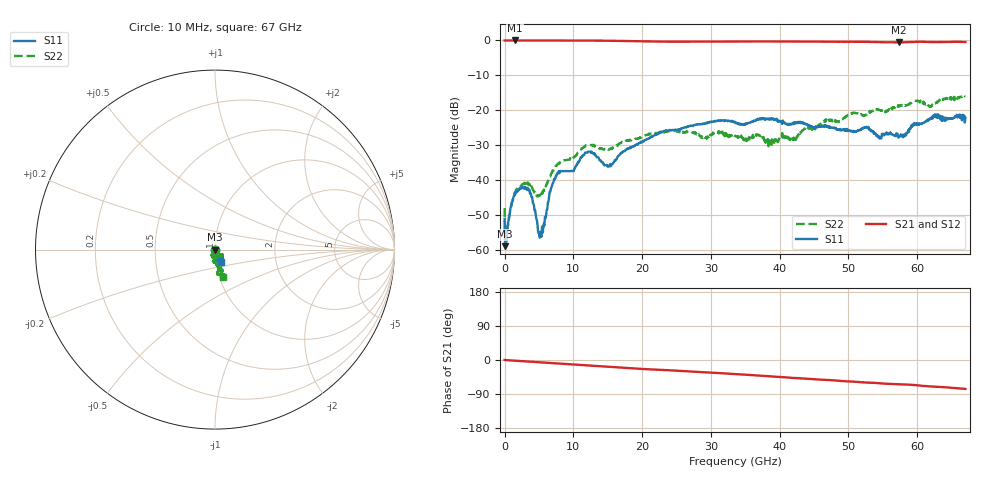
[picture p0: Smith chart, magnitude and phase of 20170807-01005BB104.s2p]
# MHz S RI R 50
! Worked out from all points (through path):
!   801 points, 10 MHz to 67 GHz, reference 50 ohm
!   highest |S21| = 0.00 dB at 1.517 GHz (marker M1); lowest = -0.6 dB at 57.37 GHz (marker M2)
!   group delay of S21, straight-line fit = 3.09 ps
!   lowest |S11| = -59.0 dB at 93.74 MHz (marker M3), VSWR 1.00, Z = 49.9 - j0.0382 ohm
!   |S11| at or under -10 dB: start of sweep to end of sweep
!   |S22| runs from -58.7 to -15.7 dB; largest |S21 - S12| = 0.021
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10  -0.000475 -0.00271  1 0.00282  1 0.00244  -0.00133 -0.00369
93.737  -0.00105 -0.000383  1 -0.00234  1 -0.00244  -0.00107 -0.000459
428.688  -0.00107 -0.00186  1 -0.00921  1 -0.00939  -0.00106 -0.00185
1014.85  -0.00119 -0.0042  1 -0.021  1 -0.021  -0.00075 -0.00451
1517.275  -0.0013 -0.00595  1 -0.031  1 -0.031  -0.00102 -0.00656
3526.975  -0.00122 -0.00701  0.997 -0.072  0.997 -0.073  0.0011 -0.00846
5285.462  -0.00157 -0.000216  0.994 -0.109  0.993 -0.108  0.00521 -0.00342
6876.475  -0.00265 -0.00755  0.989 -0.139  0.989 -0.14  0.00611 -0.011
7546.375  -0.0029 -0.011  0.987 -0.153  0.986 -0.154  0.006 -0.015
9891.025  -0.00305 -0.013  0.977 -0.2  0.977 -0.201  0.00829 -0.019
11230.83  -0.00534 -0.021  0.97 -0.228  0.97 -0.227  0.0089 -0.027
12570.62  -0.00413 -0.024  0.962 -0.256  0.962 -0.254  0.00967 -0.03
15333.96  0.00503 -0.016  0.941 -0.309  0.941 -0.31  0.018 -0.021
17511.14  0.00966 -0.024  0.919 -0.352  0.92 -0.348  0.021 -0.029
22367.91  0.038 -0.028  0.868 -0.421  0.867 -0.423  0.038 -0.027
33505  0.023 -0.064  0.769 -0.582  0.769 -0.582  -0.000348 -0.043
38696.72  0.024 -0.072  0.705 -0.662  0.706 -0.661  -0.021 -0.031
44725.82  0.013 -0.056  0.614 -0.742  0.622 -0.735  -0.000756 -0.052
55862.91  0.024 -0.038  0.43 -0.839  0.432 -0.838  0.026 -0.1
57370.19  0.019 -0.037  0.409 -0.842  0.405 -0.846  0.025 -0.11
62645.65  0.02 -0.077  0.318 -0.892  0.315 -0.893  0.012 -0.124
67000  0.036 -0.069  0.226 -0.924  0.224 -0.924  0.042 -0.152
